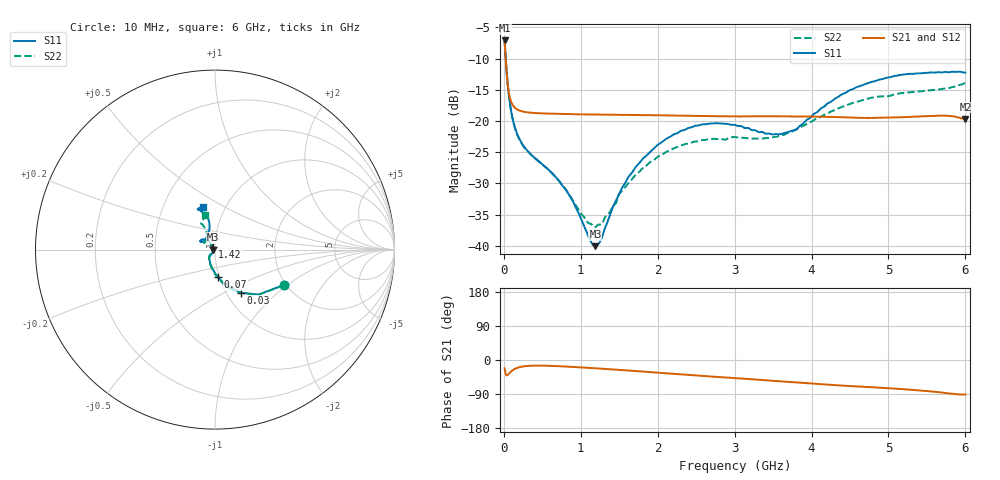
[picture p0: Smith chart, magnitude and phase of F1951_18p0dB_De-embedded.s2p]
! Integrated Device Technology
! Corporate Headquarters
! 6024 Silver Creek Valley Road
! San Jose, CA 95138  USA
! Phone:  1-408-284-8200
! Toll Free:  1-800-223-1366
! Webpage:  http://www.idt.com/
! Timing and RF Division
! 515 Groton Road, Suite 102
! Westford, MA 01886-6024
! Device:  F1951
! Description: 6-bit 0.5 dB Digital Step Attenuator
! Frequency:  100.0 -  4000.00 MHz
! Package:  4x4 mm Thin QFN Plastic Package: 24 pin
! Ports:  2 RF, 6 DC
!  Pin  1  = NC
!  Pin  2  = RF1  =  Port 1
!  Pin  3  = GND
!  Pin  4  = NC
!  Pin  5  = Serial Data Out (SDO)
!  Pin  6  = NC
!  Pin  7  = Reset Bar ( RSTb)
!  Pin  8  = Clock (CLK)
!  Pin  9  = Chip Select Bar (CSb)
!  Pin 10  = NC
!  Pin 11  = Serial Data In (SDI)
!  Pin 12  = NC
!  Pin 13  = NC
!  Pin 14  = VDD
!  Pin 15  = NC
!  Pin 16  = GND
!  Pin 17  = RF2  =  Port 2
!  Pin 18  = NC
!  Pin 19  = GND
!  Pin 20  = GND
!  Pin 21  = GND
!  Pin 22  = GND
!  Pin 23  = GND
!  Pin 24  = GND
! State:  36
! Atten State:  18.0 dB
! Voltage:  +3.30 Volts
! Current:  0.477 mA
! Data:  The device was measured on a F195X evaluation board which has
!  individual transmission lines to the RF pins.  Data was collected
!  de-embedded using a Automatic Fixture Removal [AFR] (Keysight Technologies).
!  The reference plane is the edge of the package pin.
! Misc:  Lot Code  1225BCA
!  Action Tracker AT0399
! Date Measured:  2018-09-13
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# GHz S dB R 50
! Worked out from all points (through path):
!   600 points, 10 MHz to 6 GHz, reference 50 ohm
!   highest |S21| = -7.09 dB at 10 MHz (marker M1); lowest = -19.7 dB at 6 GHz (marker M2)
!   group delay of S21, straight-line fit = 36.3 ps
!   lowest |S11| = -40.1 dB at 1.19 GHz (marker M3), VSWR 1.02, Z = 49 + j0.0334 ohm
!   |S11| at or under -10 dB: 24.51 MHz to end of sweep
!   |S22| runs from -37.0 to -7.3 dB; largest |S21 - S12| = 0.0003
!   S11 on the Smith chart (normalised r, x): 10 MHz: 1.95, -0.94; 30 MHz: 1.17, -0.61; 70 MHz: 0.98, -0.31; 1.42 GHz: 0.98, +0.03; 6 GHz: 0.79, +0.40
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0.01  -7.29 -27.1  -7.09 -21.9  -7.09 -21.9  -7.28 -27.5
0.03  -11.02 -58.6  -11.22 -39.7  -11.22 -39.8  -11.06 -59.6
0.07  -16.31 -84.1  -15.79 -35.3  -15.79 -35.3  -16.40 -85.9
0.14  -20.88 -104.2  -17.84 -23.8  -17.83 -23.8  -20.94 -106.4
0.24  -23.69 -117.7  -18.47 -17.4  -18.47 -17.3  -23.80 -120.9
0.72  -29.63 -126.6  -18.86 -16.4  -18.85 -16.4  -29.68 -136.3
0.87  -32.31 -128.4  -18.90 -18.0  -18.90 -18.0  -32.18 -140.4
1.01  -35.88 -136.1  -18.94 -19.7  -18.94 -19.7  -34.97 -149.3
1.13  -39.32 -160.0  -18.95 -21.0  -18.95 -21.0  -36.50 -166.8
1.19  -40.08 178.0  -18.96 -21.8  -18.96 -21.8  -37.03 180.0
1.26  -39.11 153.1  -18.96 -22.8  -18.96 -22.7  -36.61 166.9
1.42  -33.74 126.8  -18.99 -25.0  -18.99 -25.0  -33.62 143.5
1.64  -28.65 122.5  -19.01 -28.1  -19.02 -28.1  -29.70 133.0
2.01  -23.75 129.1  -19.09 -33.6  -19.09 -33.6  -25.66 134.9
2.49  -20.77 141.7  -19.18 -40.6  -19.18 -40.6  -23.29 142.7
3.01  -20.65 151.3  -19.26 -47.9  -19.26 -47.9  -22.58 146.7
3.59  -22.13 131.1  -19.25 -56.2  -19.25 -56.2  -22.31 129.1
3.79  -21.45 116.7  -19.29 -59.1  -19.29 -59.0  -21.39 122.3
4.01  -19.11 106.8  -19.29 -62.2  -19.29 -62.2  -20.03 116.9
4.49  -15.10 102.4  -19.44 -68.7  -19.44 -68.7  -17.32 115.1
5.01  -13.01 109.5  -19.46 -74.5  -19.46 -74.5  -15.99 117.8
6  -12.24 105.3  -19.67 -90.8  -19.67 -90.8  -13.91 106.8
